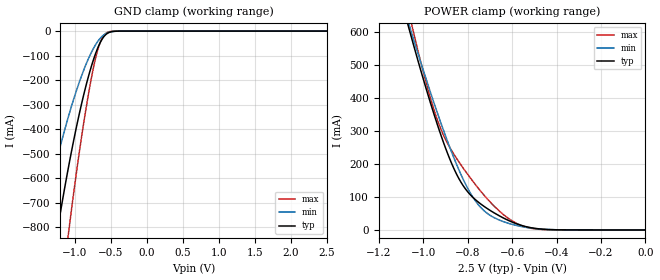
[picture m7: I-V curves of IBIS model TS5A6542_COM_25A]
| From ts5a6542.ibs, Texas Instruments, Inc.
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[Model]   TS5A6542_COM_25A
Model_type  Terminator
| variable   typ   min   max
C_comp   93.09pF   73.65pF   115.73pF
| C_tri-state   93.09pF   73.65pF   115.73pF
[Temperature Range]   40   100   -40
| Ambient temperature   25   85   -40
[Voltage range]   2.5   2.25   2.75
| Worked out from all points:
|   GND clamp passes 1 mA (typ) near -0.45 V on its own axis
|   POWER clamp passes 1 mA (typ) near -0.42 V on its own axis
[GND Clamp]
| TS5A6542_COM_25A
|   Voltage   I(typ)   I(min)   I(max)
-2.5V     -3.68A     -2.547A    -5.056A
-1.475V   -1.257A    -813.4mA   -1.841A
-1.255V   -835.4mA   -531.1mA   -1.239A
-1.23V    -791mA     -501.8mA   -1.174A
-1.085V   -549.4mA   -344.3mA   -816.2mA
-915mV    -306.9mA   -189mA     -447.4mA
-765mV    -138.1mA   -83.52mA   -182.6mA
-710mV    -89.83mA   -54.4mA    -107.3mA
-660mV    -54.07mA   -33.49mA   -55.67mA
-560mV    -11.59mA   -8.669mA   -7.174mA
-380mV    -136.1uA   -194.7uA   -18.6uA
2.5V      4.87nA     17.39uA    2.659nA
[POWER Clamp]
| TS5A6542_COM_25A
|   Voltage   I(typ)   I(min)   I(max)
-2.5V     5.061A     4.525A     6.066A
-1.075V   637.4mA    647.4mA    689.8mA
-1.06V    600.5mA    614.2mA    645.8mA
-1.045V   564.1mA    581.3mA    602.7mA
-970mV    390.7mA    422.4mA    405.3mA
-910mV    267.5mA    304.3mA    289mA
-820mV    134mA      153.3mA    187.4mA
-770mV    94.76mA    92.67mA    141.7mA
-715mV    66.3mA     51.94mA    96.66mA
-615mV    28.43mA    19.87mA    34.27mA
-515mV    6.782mA    5.677mA    5.198mA
-31.15fV  4.87nA     19.15nA    2.945nA
